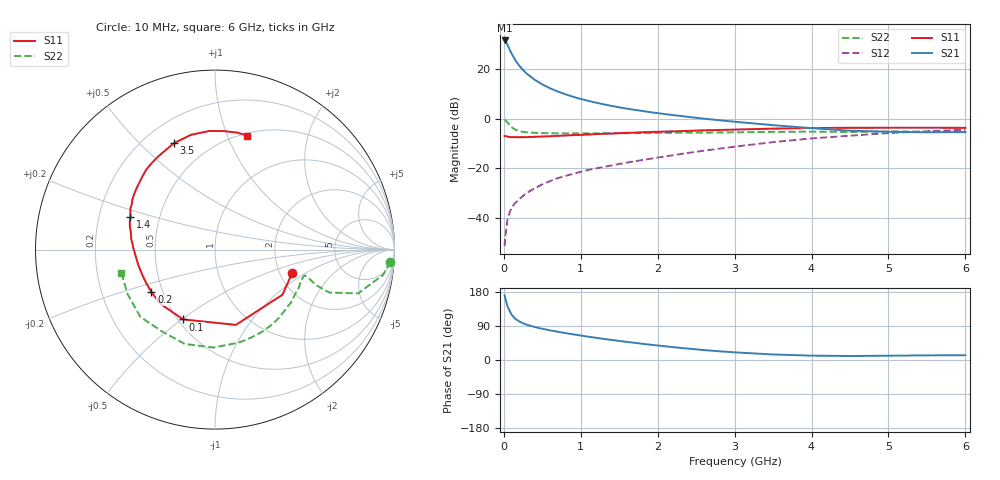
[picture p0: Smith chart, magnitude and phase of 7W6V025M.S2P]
! Infineon Technologies  Discrete & RF Semiconductors
! BFS17W
! Si NPN RF Bipolar Junction Transistor in SOT323
! VCE = 6 V  IC = 25 mA
! Common Emitter S-Parameters:  August  1999
# GHz  S  MA  R  50
!  f  S11  S21  S12  S22
! GHz  MAG  ANG  MAG  ANG  MAG  ANG  MAG  ANG
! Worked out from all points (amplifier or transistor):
!   36 points, 10 MHz to 6 GHz, reference 50 ohm
!   highest |S21| = 31.6 dB at 10 MHz (marker M1)
!   |S21| within 3 dB of that: start of sweep to 65.88 MHz
!   unconditionally stable (mu >= 1): 257.8 MHz to 2.048 GHz; 5.326 GHz to end of sweep
!   at 250 MHz: K = 0.99, MSG = 25.4 dB, |S12| = -31.1 dB
!   at 1.4 GHz: K = 1.16, MAG = 9.6 dB, |S12| = -18.8 dB
!   at 6 GHz: K = 1.04, MAG = -1.7 dB, |S12| = -4.4 dB
!   S11 on the Smith chart (normalised r, x): 10 MHz: 2.33, -0.77; 100 MHz: 0.53, -0.51; 200 MHz: 0.43, -0.25; 1.4 GHz: 0.34, +0.16; 3.5 GHz: 0.32, +0.64; 6 GHz: 0.53, +1.18
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0.01  0.449 -17.1  38.23 171.0  0.0027 80.2  0.9777 -3.9
0.02  0.4523 -33.8  37.18 161.9  0.0043 78.8  0.9476 -8.5
0.05  0.4353 -74.5  30.55 140.4  0.0101 69.1  0.8345 -17.0
0.1  0.4275 -114.5  20.86 119.8  0.0161 61.4  0.6811 -20.6
0.15  0.4286 -135.0  15.23 108.6  0.0202 60.5  0.6042 -19.5
0.2  0.4263 -146.2  11.86 101.8  0.024 63.9  0.5681 -18.1
0.25  0.4261 -154.2  9.659 96.9  0.0279 64.7  0.5461 -16.9
0.3  0.4282 -159.5  8.13 93.1  0.0322 66.4  0.5355 -16.4
0.4  0.435 -167.8  6.17 87.1  0.0398 68.2  0.5218 -16.1
0.5  0.4402 -173.0  4.966 82.4  0.0477 70.2  0.5173 -16.5
0.6  0.4462 -177.1  4.14 78.3  0.0555 70.8  0.5139 -17.5
0.7  0.4543 179.4  3.572 74.6  0.0636 71.4  0.5115 -18.9
0.9  0.4704 172.8  2.792 67.8  0.0778 72.6  0.5101 -22.3
1.1  0.4836 166.8  2.304 61.4  0.0933 72.9  0.5112 -26.3
1.4  0.5044 159.0  1.826 53.0  0.1144 73.6  0.5148 -33.1
1.8  0.5367 149.2  1.442 42.8  0.1476 74.8  0.5172 -43.2
2.2  0.5596 139.9  1.192 33.9  0.1849 74.8  0.5242 -53.6
2.8  0.5969 126.2  0.939 23.0  0.2503 72.4  0.5314 -70.5
3.5  0.6355 111.2  0.747 14.6  0.3394 66.6  0.5458 -91.0
4.5  0.6616 92.7  0.577 10.5  0.4577 53.8  0.5433 -123.3
5.5  0.6634 79.2  0.536 12.3  0.5622 40.6  0.5469 -153.0
6  0.66 74.1  0.544 12.6  0.6035 34.1  0.5374 -166.2
